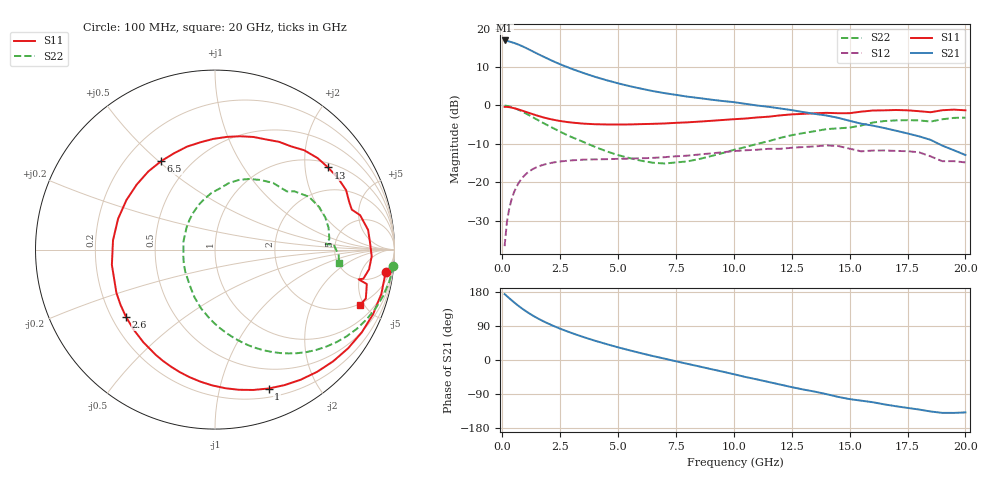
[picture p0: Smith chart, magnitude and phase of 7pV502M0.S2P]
! Infineon Technologies  Discrete & RF Semiconductors
! bfp620
! VCE = 0.50 V,  IC =  2.0 mA
! Common Emitter S-Parameters:  Sep 2002
# GHz  S  MA  R  50
!  f  S11  S21  S12  S22
! GHz  MAG  ANG  MAG  ANG  MAG  ANG  MAG  ANG
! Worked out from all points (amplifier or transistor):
!   59 points, 100 MHz to 20 GHz, reference 50 ohm
!   highest |S21| = 16.9 dB at 100 MHz (marker M1)
!   |S21| within 3 dB of that: start of sweep to 1.368 GHz
!   unconditionally stable (mu >= 1): 5.786 GHz to 12.27 GHz; 14.64 GHz to 15.65 GHz; 17.09 GHz to end of sweep
!   at 1 GHz: K = 0.19, MSG = 16.5 dB, |S12| = -18.0 dB
!   at 5.5 GHz: K = 0.96, MSG = 9.4 dB, |S12| = -13.8 dB
!   at 20 GHz: K = 2.00, MAG = -4.8 dB, |S12| = -14.8 dB
!   S11 on the Smith chart (normalised r, x): 100 MHz: 4, -14; 1 GHz: 0.29, -1.42; 2.6 GHz: 0.26, -0.32; 6.5 GHz: 0.35, +0.51; 13 GHz: 1.14, +2.64; 20 GHz: 1.92, -4.69
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0.1  0.9593 -7.5  7.011 173.8  0.0148 84.3  0.9971 -5.3
0.3  0.9514 -22.2  6.792 163.1  0.0457 76.6  0.9724 -15.3
0.6  0.9059 -43.4  6.362 147.6  0.086 63.9  0.905 -29.2
0.8  0.8682 -56.6  6.016 138.2  0.1081 56.1  0.8503 -37.4
1  0.8295 -68.9  5.641 129.6  0.1265 49.2  0.7928 -44.9
1.4  0.7567 -91.2  4.907 114.3  0.1533 37.6  0.6811 -57.8
1.8  0.697 -110.5  4.284 101.4  0.1702 28.6  0.5852 -68.4
2.2  0.6528 -127.6  3.763 90.2  0.1813 21.3  0.5067 -77.5
2.6  0.6218 -142.8  3.339 80.2  0.1884 15.2  0.4405 -86.1
3  0.5996 -156.4  2.994 71.1  0.1933 9.9  0.3877 -94.1
3.5  0.5808 -171.6  2.649 60.6  0.1975 4.4  0.336 -103.5
4  0.5706 174.8  2.361 50.9  0.199 -0.4  0.2898 -113.1
5  0.5654 150.8  1.943 33.4  0.2021 -7.3  0.2263 -131.8
6.5  0.577 121.3  1.54 10.5  0.2083 -15.4  0.1802 -168.1
7  0.5836 112.8  1.449 3.7  0.2126 -17.6  0.1759 179.3
8.5  0.6169 90.9  1.249 -16.9  0.2303 -25.0  0.2011 141.8
10.5  0.6768 65.0  1.051 -44.8  0.2615 -39.4  0.2877 102.0
13  0.7784 36.0  0.821 -77.9  0.2883 -59.6  0.4376 64.1
13.5  0.7925 30.3  0.777 -83.5  0.2938 -64.3  0.4634 56.8
15  0.794 16.3  0.632 -103.2  0.2744 -84.7  0.5159 38.9
17  0.8738 -2.5  0.47 -122.0  0.2565 -96.0  0.6401 16.2
20  0.8654 -20.8  0.227 -138.3  0.1818 -115.8  0.6957 -6.3
